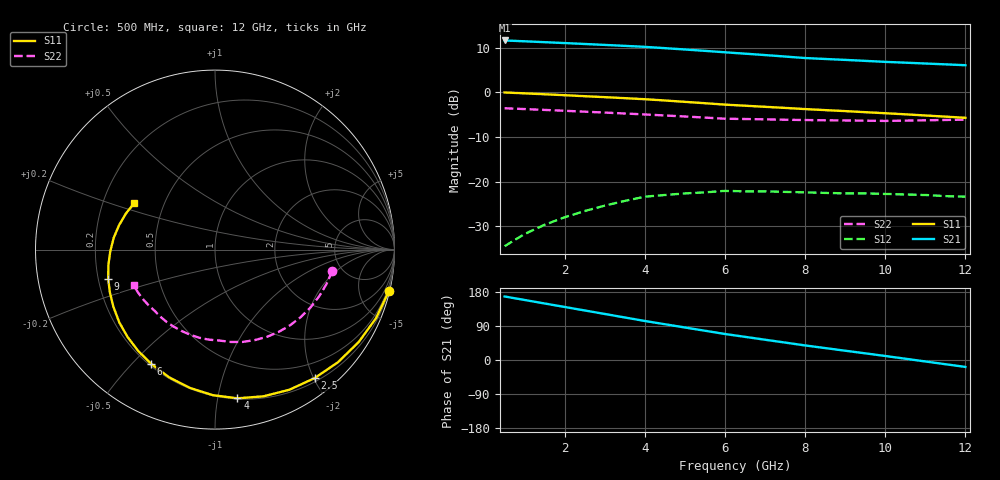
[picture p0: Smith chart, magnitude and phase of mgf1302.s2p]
! MGF1302  (Ta=25deg. C, VDS=3V, lDS=10mA)
! From 1996/1997 GaAs FET/MMIC Data book
# GHZ S MA R 50
!  Freq.  S11  S21  S12  S22
!  GHz  (mag)  (ang)  (mag)  (ang)  (mag)  (ang)  (mag)  (ang)
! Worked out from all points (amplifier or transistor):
!   24 points, 500 MHz to 12 GHz, reference 50 ohm
!   highest |S21| = 11.6 dB at 500 MHz (marker M1)
!   |S21| within 3 dB of that: start of sweep to 6.569 GHz
!   unconditionally stable (mu >= 1): 7.087 GHz to end of sweep
!   at 2.5 GHz: K = 0.40, MSG = 18.7 dB, |S12| = -26.6 dB
!   at 6.5 GHz: K = 0.90, MSG = 15.4 dB, |S12| = -22.2 dB
!   at 12 GHz: K = 1.95, MAG = 9.1 dB, |S12| = -23.3 dB
!   lowest NFmin = 0.96 dB at 4 GHz
!   S11 on the Smith chart (normalised r, x): 500 MHz: 0.11, -8.58; 2.5 GHz: 0.25, -2.02; 4 GHz: 0.21, -1.14; 6 GHz: 0.21, -0.57; 9 GHz: 0.24, -0.13; 12 GHz: 0.34, +0.24
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0.5  0.997 -13.3  3.809 167.6  0.019 80.1  0.664 -10.3
1  0.975 -23.1  3.727 158.4  0.026 73.1  0.65 -17.3
1.5  0.952 -32.8  3.644 149.1  0.033 66.0  0.636 -24.2
2  0.929 -42.5  3.561 139.9  0.04 58.9  0.622 -31.2
2.5  0.906 -52.2  3.478 130.7  0.047 51.8  0.608 -38.2
3  0.884 -62.0  3.396 121.5  0.054 44.8  0.594 -45.2
3.5  0.861 -71.7  3.313 112.2  0.061 37.7  0.58 -52.1
4  0.838 -81.4  3.23 103.0  0.068 30.6  0.566 -59.1
4.5  0.811 -90.9  3.124 94.4  0.071 24.5  0.551 -66.2
5  0.783 -100.3  3.018 85.8  0.074 18.5  0.537 -73.3
5.5  0.756 -109.8  2.913 77.2  0.076 12.4  0.522 -80.3
6  0.729 -119.2  2.807 68.6  0.079 6.3  0.507 -87.4
6.5  0.709 -127.0  2.71 61.1  0.078 1.1  0.503 -93.7
7  0.689 -134.9  2.614 53.5  0.078 -4.1  0.499 -100.1
7.5  0.67 -142.7  2.517 46.0  0.077 -9.2  0.494 -106.4
8  0.65 -150.5  2.421 38.4  0.076 -14.4  0.49 -112.7
8.5  0.633 -157.6  2.364 31.5  0.075 -18.1  0.487 -118.2
9  0.617 -164.7  2.308 24.5  0.074 -21.9  0.485 -123.7
9.5  0.6 -171.8  2.251 17.6  0.074 -25.6  0.482 -129.2
10.5  0.568 173.3  2.149 3.4  0.072 -33.9  0.483 -140.1
11  0.551 165.5  2.103 -3.9  0.071 -38.4  0.487 -145.5
12  0.519 149.9  2.012 -18.3  0.068 -47.5  0.495 -156.2
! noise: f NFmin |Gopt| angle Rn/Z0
4  0.96  0.595  63.5  0.55
8  1.85  0.475  134.5  0.6
12  2.76  0.385  -155.3  0.3
